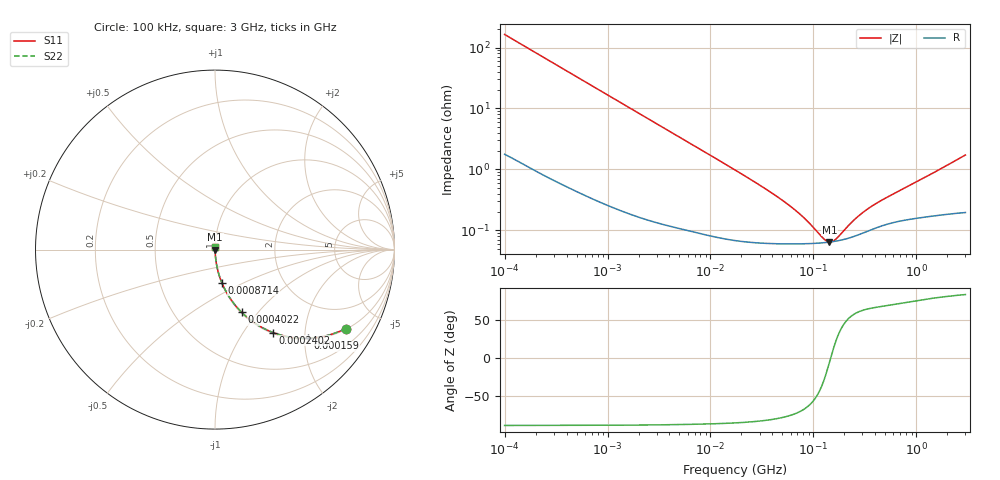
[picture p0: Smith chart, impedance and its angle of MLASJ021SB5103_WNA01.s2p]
! MLASJ021SB5103_WNA01  S-PARAMETER MODEL  ( Standard Model )
! Model Generated by TAIYO YUDEN Corporation (http://www.ty-top.com)
! Version 1.0
! TAIYO YUDEN Control No. 220901
! Copyright(c) 2022 TAIYO YUDEN CO.,LTD. All Rights Reserved.
! Product Description (link to TY-COMPAS)
! https://ds.yuden.co.jp/TYCOMPAS/or/detail?pn=MLASJ021SB5103KWNA01&u=M
! Products Name : Multilayer Ceramic Capacitors
! Characteristics :
!  Capacitance : 0.01 [uF] , Rated Voltage : 6.3 [V] , TCC : X5R
!  Case Size : 0.25 x 0.125 / 0.0098 x 0.0049 [mm/inch] , Thickness : 0.125 / 0.0049 [mm/inch]
!  (Conditions: Temperature = 25 [degC] , DC Bias Voltage = 0 [V])
! External Node Assignments :
!  1  o---| |---o  2
! GND o---------o GND
! Frequency Range : 100kHz  -  3GHz  [ 401 STEP ]
# MHZ S RI R 50
! Freq[MHz].  S11 Real  S11 Imag  S21 Real  S21 Imag  S12 Real  S12 Imag  S22 Real  S22 Imag
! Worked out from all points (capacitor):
!   401 points, 100 kHz to 3 GHz, reference 50 ohm
!   read as one part in series: C = 9.67 nF near 105.3 kHz
!   lowest |Z| = 64.3 mohm at 143.3 MHz (marker M1)
!   series resonance near 147.5 MHz, so ESL is about 120 pH
!   S11 on the Smith chart (normalised r, x): 100 kHz: 1.04, -3.28; 159 kHz: 1.02, -2.07; 240.2 kHz: 1.02, -1.38; 402.2 kHz: 1.01, -0.82; 871.4 kHz: 1.01, -0.38; 3 GHz: 1.00, +0.03
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0.1  0.7274 -0.4399  0.2726 0.4399  0.2726 0.4399  0.7274 -0.4399
0.159027  0.5178 -0.4941  0.4822 0.4941  0.4822 0.4941  0.5178 -0.4941
0.24019  0.3234 -0.462  0.6766 0.462  0.6766 0.462  0.3234 -0.462
0.310802  0.2239 -0.4109  0.7761 0.4109  0.7761 0.4109  0.2239 -0.4109
0.402172  0.1485 -0.3494  0.8515 0.3494  0.8515 0.3494  0.1485 -0.3494
0.562235  0.0835 -0.27  0.9165 0.27  0.9165 0.27  0.0835 -0.27
0.871356  0.0379 -0.1837  0.9621 0.1837  0.9621 0.1837  0.0379 -0.1837
1.576268  0.013 -0.1047  0.987 0.1047  0.987 0.1047  0.013 -0.1047
3.161081  0.00412 -0.053  0.9959 0.053  0.9959 0.053  0.00412 -0.053
17.7727  0.000763 -0.0095  0.9992 0.0095  0.9992 0.0095  0.000763 -0.0095
33.85116  0.000633 -0.00481  0.9994 0.00481  0.9994 0.00481  0.000633 -0.00481
52.46276  0.000605 -0.00287  0.9994 0.00287  0.9994 0.00287  0.000605 -0.00287
73.34282  0.000601 -0.00177  0.9994 0.00177  0.9994 0.00177  0.000601 -0.00177
97.38194  0.000607 -0.000998  0.9994 0.000998  0.9994 0.000998  0.000607 -0.000998
126.0104  0.000624 -0.000369  0.9994 0.000369  0.9994 0.000369  0.000624 -0.000369
143.341  0.000639 -6.61e-05  0.9994 6.61e-05  0.9994 6.61e-05  0.000639 -6.61e-05
154.8634  0.00065 0.000114  0.9993 -0.000114  0.9993 -0.000114  0.00065 0.000114
167.3121  0.000665 0.000295  0.9993 -0.000295  0.9993 -0.000295  0.000665 0.000295
240.0085  0.000778 0.00116  0.9992 -0.00116  0.9992 -0.00116  0.000778 0.00116
310.5665  0.000916 0.00181  0.9991 -0.00181  0.9991 -0.00181  0.000916 0.00181
547.5153  0.0013 0.00341  0.9987 -0.00341  0.9987 -0.00341  0.0013 0.00341
3000  0.00224 0.017  0.9978 -0.017  0.9978 -0.017  0.00224 0.017
